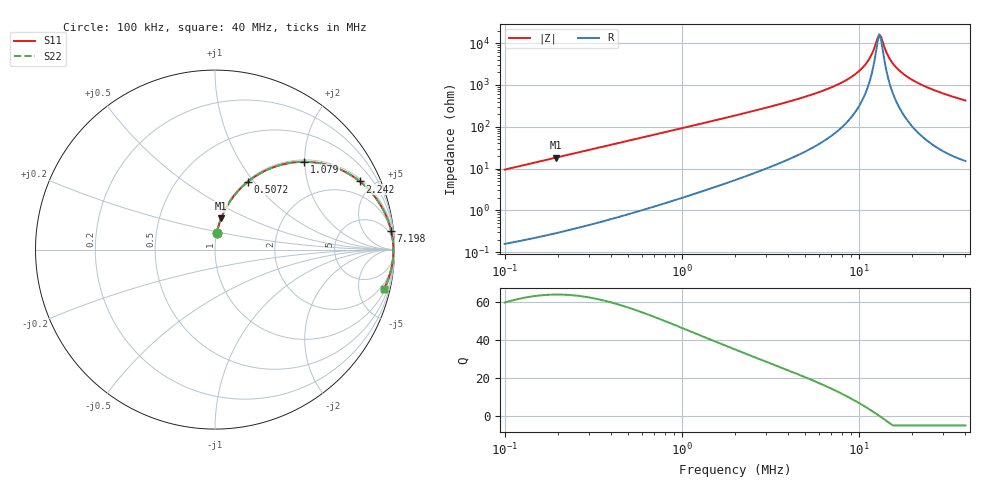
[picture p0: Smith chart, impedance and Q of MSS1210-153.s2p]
# MHz S MA R 50
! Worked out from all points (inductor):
!   263 points, 100 kHz to 40 MHz, reference 50 ohm
!   read as one part in series: L = 15 uH near 102.3 kHz
!   highest Q = 64.1 at 194.1 kHz (marker M1), where L = 14.9 uH
!   self-resonance near 13.04 MHz
!   S11 on the Smith chart (normalised r, x): 100 kHz: 1.00, +0.19; 507.2 kHz: 1.02, +0.94; 1.079 MHz: 1.04, +1.99; 2.242 MHz: 1.13, +4.18; 7.198 MHz: 2, +18; 40 MHz: 1.30, -8.50
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0.1  0.0937 83.7  0.994 -5.4  0.994 -5.4  0.0937 83.7
0.194095  0.178 78.9  0.9812 -10.3  0.9812 -10.3  0.178 78.9
0.2735188  0.2458 74.9  0.9654 -14.2  0.9654 -14.2  0.2458 74.9
0.5071523  0.4217 64.1  0.8994 -24.9  0.8994 -24.9  0.4217 64.1
0.7481253  0.5625 54.7  0.8159 -34.2  0.8159 -34.2  0.5625 54.7
1.078646  0.6969 44.6  0.7019 -44.2  0.7019 -44.2  0.6969 44.6
2  0.8702 27.9  0.4685 -60.4  0.4685 -60.4  0.8702 27.9
2.242269  0.8919 25.2  0.4263 -63.1  0.4263 -63.1  0.8919 25.2
5.470376  0.9777 9.5  0.1647 -77.5  0.1647 -77.5  0.9777 9.5
7.197729  0.9866 6.1  0.1072 -79.7  0.1072 -79.7  0.9866 6.1
9.047128  0.991 3.7  0.06447 -80.1  0.06447 -80.1  0.991 3.7
10.61772  0.9928 2.1  0.03648 -77.6  0.03648 -77.6  0.9928 2.1
11.37172  0.9933 1.4  0.0249 -73.7  0.0249 -73.7  0.9933 1.4
11.90389  0.9936 0.9  0.01741 -67.9  0.01741 -67.9  0.9936 0.9
13.04413  0.9939 0.0  0.006157 -5.8  0.006157 -5.8  0.9939 0.0
13.34586  0.9939 -0.2  0.006913 28.1  0.006913 28.1  0.9939 -0.2
14.29359  0.9939 -0.9  0.01615 67.4  0.01615 67.4  0.9939 -0.9
14.96251  0.9938 -1.3  0.02361 74.2  0.02361 74.2  0.9938 -1.3
17.16301  0.9931 -2.7  0.04713 80.3  0.04713 80.3  0.9931 -2.7
20.60847  0.991 -4.6  0.08022 81.3  0.08022 81.3  0.991 -4.6
27.1159  0.9847 -7.7  0.1348 79.6  0.1348 79.6  0.9847 -7.7
40  0.9658 -13.1  0.2272 74.8  0.2272 74.8  0.9658 -13.1
